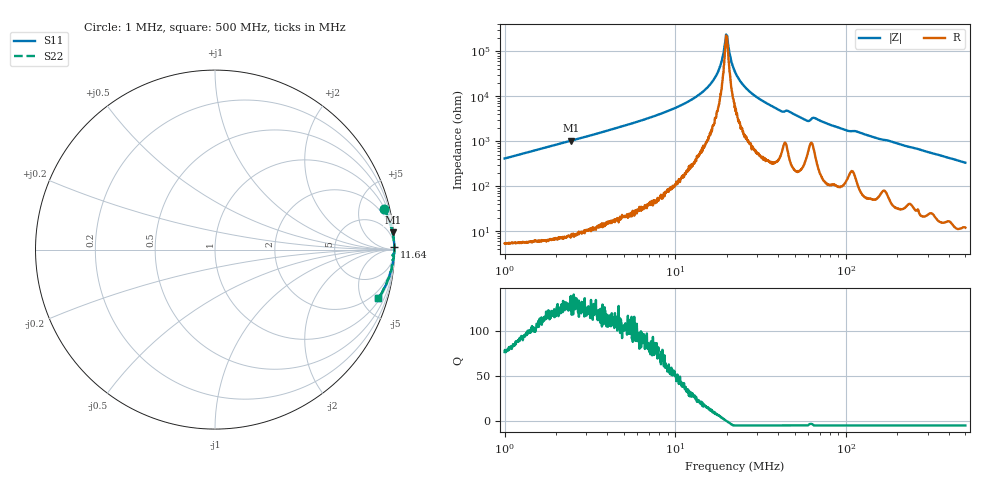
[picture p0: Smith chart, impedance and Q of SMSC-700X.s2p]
!s-Parameter Generated by FASTRON Sdn. Bhd.
!FASTRON P/N : SMSC-700X
!Keysight Technologies,E4991B,MY54100416,A.01.15
!Date: Thu Mar 19 13:12:31 2026
!Version  : Rev00 Thu Mar 19 13:12:31 2026
!Data & Calibration Information:
!PortZ  Port1:50+j0  Port2:50+j0
!When reading, reference impedance value at option line is always used.
! Remarks : This data is being provided solely for informational purposes.
!Freq	S11	S21	S12	S22
# Hz S dB R 50
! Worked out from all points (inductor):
!   1601 points, 1 MHz to 500 MHz, reference 50 ohm
!   read as one part in series: L = 65.8 uH near 1.032 MHz
!   highest Q = 132 at 2.462 MHz (marker M1), where L = 66.7 uH
!   self-resonance near 19.9 MHz
!   S11 on the Smith chart (normalised r, x): 1 MHz: 1.11, +8.28; 11.64 MHz: open; 500 MHz: 1.24, -6.69
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1000000  -0.27 13.5  -12.62 -75.7  -12.62 -75.7  -0.27 13.5
2462355  -0.05 5.5  -20.32 -84.0  -20.32 -84.0  -0.05 5.5
2820919  -0.04 4.8  -21.54 -84.8  -21.54 -84.8  -0.04 4.8
7957584  -0.01 1.5  -31.85 -87.8  -31.85 -87.8  -0.01 1.5
1.164376e7  -0.00 0.8  -37.25 -87.6  -37.25 -87.6  -0.00 0.8
1.452928e7  -0.00 0.5  -42.06 -86.5  -42.06 -86.5  -0.00 0.5
1.690563e7  -0.00 0.2  -47.91 -84.1  -47.91 -84.1  -0.00 0.2
1.827126e7  -0.00 0.1  -53.22 -78.3  -53.22 -78.3  -0.00 0.1
1.951844e7  -0.00 0.0  -63.57 -48.6  -63.57 -48.6  -0.00 0.0
1.982405e7  -0.00 0.0  -67.48 -20.1  -67.48 -20.1  -0.00 0.0
2.029147e7  -0.00 -0.0  -64.46 45.1  -64.46 45.1  -0.00 -0.0
2.134237e7  -0.00 -0.1  -55.00 74.7  -55.00 74.7  -0.00 -0.1
2.236068e7  -0.00 -0.2  -50.85 79.8  -50.85 79.8  -0.00 -0.2
2.561681e7  -0.00 -0.4  -44.08 85.0  -44.08 85.0  -0.00 -0.4
3.196508e7  -0.01 -0.7  -38.24 86.2  -38.24 86.2  -0.01 -0.7
4.130554e7  -0.02 -1.2  -33.58 83.2  -33.58 83.2  -0.02 -1.2
4.587261e7  -0.02 -1.2  -33.45 82.4  -33.45 82.4  -0.02 -1.2
5.836312e7  -0.05 -1.9  -29.32 80.1  -29.32 80.1  -0.05 -1.9
6.307767e7  -0.08 -1.7  -30.25 71.9  -30.25 71.9  -0.08 -1.7
1.005306e8  -0.05 -3.3  -24.89 82.4  -24.89 82.4  -0.05 -3.3
1.77937e8  -0.08 -5.5  -20.31 81.5  -20.31 81.5  -0.08 -5.5
5e8  -0.46 -16.5  -10.94 71.5  -10.94 71.5  -0.46 -16.5
